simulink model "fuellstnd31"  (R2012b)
settings: Solver=ode45  StartTime=0.0  StopTime=10.0  RelTol=1e-3
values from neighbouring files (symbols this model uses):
  A1 = 0.02    [fuellstnd_1.m]    (also in fuellstnd_2.m; fuellstnd_21.m; fuellstnd_3.m; fuellstnd_31.m)
  A12 = 0.005    [fuellstnd_1.m]    (also in fuellstnd_2.m; fuellstnd_21.m; fuellstnd_3.m; fuellstnd_31.m)
  A2 = A1    (= 0.02)    [fuellstnd_1.m]    (also in fuellstnd_2.m; fuellstnd_21.m; fuellstnd_3.m; fuellstnd_31.m)
  A23 = A12    (= 0.005)    [fuellstnd_1.m]    (also in fuellstnd_2.m; fuellstnd_21.m; fuellstnd_3.m; fuellstnd_31.m)
  A3 = A1    (= 0.02)    [fuellstnd_1.m]    (also in fuellstnd_2.m; fuellstnd_21.m; fuellstnd_3.m; fuellstnd_31.m)
  A30 = A12    (= 0.005)    [fuellstnd_1.m]    (also in fuellstnd_2.m; fuellstnd_21.m; fuellstnd_3.m; fuellstnd_31.m)
  g = 9.89    [fuellstnd_1.m]    (also in fuellstnd_2.m; fuellstnd_21.m; fuellstnd_3.m; fuellstnd_31.m)
  h10 = 0.0    (= 0)    [fuellstnd_1.m]    (also in fuellstnd_2.m; fuellstnd_21.m; fuellstnd_3.m; fuellstnd_31.m)
  h20 = h10    (= 0)    [fuellstnd_1.m]    (also in fuellstnd_2.m; fuellstnd_21.m; fuellstnd_3.m; fuellstnd_31.m)
  h30 = h10    (= 0)    [fuellstnd_1.m]    (also in fuellstnd_2.m; fuellstnd_21.m; fuellstnd_3.m; fuellstnd_31.m)
  hy = 0.01    [fuellstnd_3.m]    (also in fuellstnd_31.m; regulator_1.m = 2; zweipunkt_1.m = 20; zweipunkt_2.m = 0)
  nenner_rueck = nenner_rueck{:}    [fuellstnd_3.m]    (also in fuellstnd_31.m; zweipunkt_31.m; zweipunkt_32.m)
  Tp = 1    [fuellstnd_2.m]    (also in fuellstnd_21.m = 0.1; fuellstnd_3.m = 0.1; fuellstnd_31.m = 0.01; regulator_1.m = 5)
  Ts = 0.001    [fuellstnd_3.m]    (also in fuellstnd_31.m; kalman_d1.m = 0.05; kalman_d2.m = 0.1; kalman_d3.m = 0.1)
  Usoll = 0.4,    [fuellstnd_2.m]    (also in fuellstnd_21.m = 0.2,; fuellstnd_3.m = 0.2,; fuellstnd_31.m = 0.2,)
  zaehl_rueck = zaehl_rueck{:}    [fuellstnd_3.m]    (also in fuellstnd_31.m; zweipunkt_31.m; zweipunkt_32.m)
undefined symbols (not defined in the file or in its folder): sgn

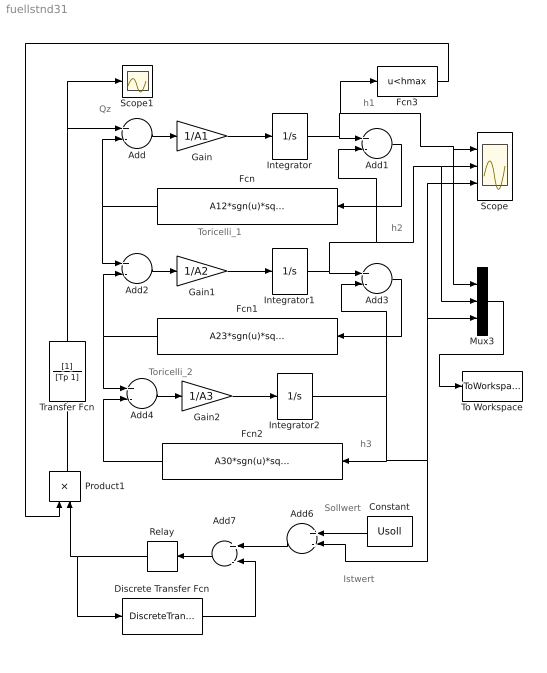
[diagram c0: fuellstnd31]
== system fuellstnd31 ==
  note: Istwert
  note: Sollwert
  note: h3
  note: h2
  note: h1
  note: Toricelli_2
  note: Toricelli_1
  note: Qz
  Add{,1..4,6..7} (7 alike) : Sum  Inputs=+-
  Constant : Constant  Value=Usoll
  Discrete Transfer Fcn : DiscreteTransferFcn  Numerator=[zaehl_rueck]  Denominator=[nenner_rueck]  SampleTime=Ts
  Fcn : Fcn  Expr=A12*sgn(u)*sqrt(2*g*abs(u))
  Fcn1 : Fcn  Expr=A23*sgn(u)*sqrt(2*g*abs(u))
  Fcn2 : Fcn  Expr=A30*sgn(u)*sqrt(2*g*abs(u))
  Fcn3 : Fcn  Expr=u<hmax
  Gain : Gain  Gain=1/A1
  Gain1 : Gain  Gain=1/A2
  Gain2 : Gain  Gain=1/A3
  Integrator : Integrator  InitialCondition=h10
  Integrator1 : Integrator  InitialCondition=h20
  Integrator2 : Integrator  InitialCondition=h30
  Mux3 : Mux  Inputs=3
  Product1 : Product
  Relay : Relay  OnSwitchValue=hy  OffSwitchValue=-hy  OnOutputValue=Qz  ZeroCross=off
  Scope : Scope  NumInputPorts=3
  Scope1 : Scope
  To Workspace : ToWorkspace  VariableName=y  SampleTime=-1  SaveFormat=Structure With Time
  Transfer Fcn : TransferFcn  Denominator=[Tp 1]
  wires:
  Add/1 -> Gain/1
  Gain/1 -> Integrator/1
  Add1/1 -> Fcn/1
  Fcn/1 -> Add2/1, Add/2
  Add2/1 -> Gain1/1
  Gain1/1 -> Integrator1/1
  Fcn1/1 -> Add4/1, Add2/2
  Add4/1 -> Gain2/1
  Gain2/1 -> Integrator2/1
  Fcn2/1 -> Add4/2
  Integrator2/1 -> Fcn2/1, Mux3/3, Scope/3, Add6/2, Add3/2
  Mux3/1 -> To Workspace/1
  Relay/1 -> Product1/2, Discrete Transfer Fcn/1
  Integrator1/1 -> Mux3/2, Scope/2, Add1/2, Add3/1
  Integrator/1 -> Fcn3/1, Mux3/1, Scope/1, Add1/1
  Constant/1 -> Add6/1
  Add3/1 -> Fcn1/1
  Add6/1 -> Add7/1
  Add7/1 -> Relay/1
  Discrete Transfer Fcn/1 -> Add7/2
  Transfer Fcn/1 -> Scope1/1, Add/1
  Fcn3/1 -> Product1/1
  Product1/1 -> Transfer Fcn/1
